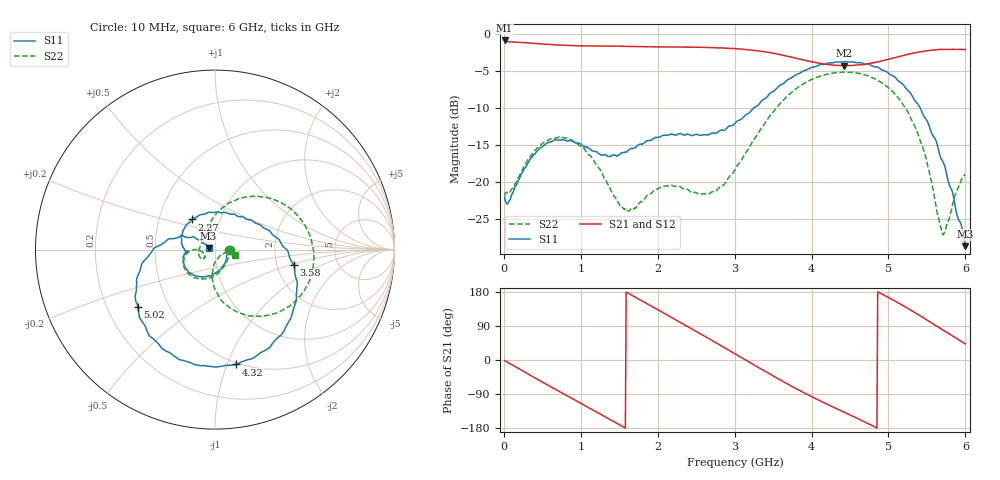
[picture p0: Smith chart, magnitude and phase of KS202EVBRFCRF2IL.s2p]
!Agilent Technologies,N5230A,MY45001650,A.07.50.48
!Agilent N5230A: A.07.50.48
!Date: Monday, June 12, 2017 12:47:22
!Correction: S11(Full 2 Port(1,2))
!S21(Full 2 Port(1,2))
!S12(Full 2 Port(1,2))
!S22(Full 2 Port(1,2))
!S2P File: Measurements: S11, S21, S12, S22:
# Hz S  dB  R 50
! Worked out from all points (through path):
!   600 points, 10 MHz to 6 GHz, reference 50 ohm
!   highest |S21| = -0.82 dB at 10 MHz (marker M1); lowest = -4.2 dB at 4.42 GHz (marker M2)
!   group delay of S21, straight-line fit = 310 ps
!   lowest |S11| = -28.7 dB at 6 GHz (marker M3), VSWR 1.08, Z = 46.6 + j0.872 ohm
!   |S11| at or under -10 dB: start of sweep to 3.242 GHz; 5.414 GHz to end of sweep
!   |S22| runs from -27.2 to -5.1 dB; largest |S21 - S12| = 0.0024
!   S11 on the Smith chart (normalised r, x): 10 MHz: 1.17, -0.00; 2.27 GHz: 0.73, +0.26; 3.58 GHz: 2.49, -0.54; 4.32 GHz: 0.49, -1.08; 5.02 GHz: 0.33, -0.30; 6 GHz: 0.93, +0.02
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1e7  -22.02 -1.4  -0.82 -1.4  -0.81 -1.4  -21.83 -0.4
2.6e8  -18.30 -80.7  -1.11 -30.5  -1.10 -30.5  -17.90 -78.6
5.4e8  -14.89 -125.5  -1.33 -62.8  -1.33 -62.8  -14.55 -121.2
7.8e8  -14.30 -150.8  -1.47 -89.7  -1.47 -89.7  -14.02 -146.7
1.01e9  -14.95 -168.0  -1.54 -115.4  -1.54 -115.3  -15.22 -166.2
1.51e9  -16.25 -175.8  -1.58 -171.8  -1.58 -171.6  -23.25 -167.6
1.75e9  -14.99 176.7  -1.65 161.2  -1.65 161.3  -23.01 -143.0
2.01e9  -13.93 156.4  -1.69 131.7  -1.69 131.8  -20.88 -147.5
2.27e9  -13.46 127.7  -1.71 102.1  -1.71 102.2  -20.55 -168.8
2.61e9  -13.60 86.8  -1.75 62.7  -1.76 62.8  -21.60 152.4
3.01e9  -11.97 41.2  -1.93 15.7  -1.93 15.9  -18.22 110.9
3.27e9  -9.82 18.5  -2.18 -15.0  -2.17 -14.9  -13.96 88.0
3.58e9  -6.95 -11.2  -2.72 -51.2  -2.71 -51.1  -9.50 60.2
4.01e9  -4.44 -51.5  -3.71 -97.7  -3.71 -97.7  -6.07 22.5
4.32e9  -3.73 -79.6  -4.19 -127.8  -4.19 -127.8  -5.18 -2.9
4.42e9  -3.70 -88.5  -4.23 -137.3  -4.23 -137.4  -5.11 -10.7
4.66e9  -3.89 -109.5  -4.07 -160.2  -4.07 -160.2  -5.39 -29.9
5.01e9  -5.34 -142.5  -3.34 163.9  -3.33 163.9  -7.32 -59.4
5.02e9  -5.44 -143.6  -3.32 162.8  -3.31 162.8  -7.40 -60.3
5.38e9  -9.40 178.4  -2.43 120.7  -2.43 120.7  -13.38 -90.9
5.7e9  -17.08 148.8  -2.03 80.2  -2.03 80.1  -26.92 -57.4
6e9  -28.69 165.3  -2.05 42.5  -2.04 42.5  -18.99 -14.1
